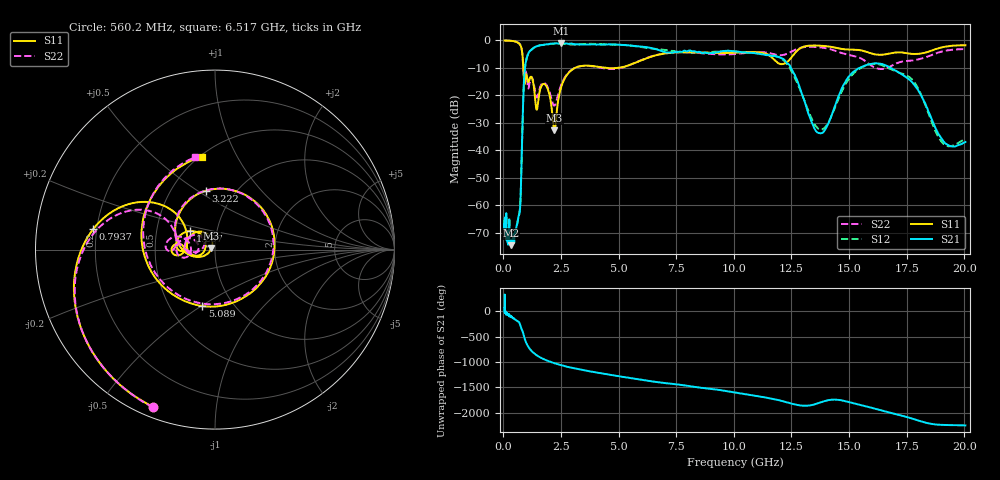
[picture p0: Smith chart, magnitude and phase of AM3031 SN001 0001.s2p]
# Hz S DB R 50
!freq MagS11 AngS11 MagS21 AngS21 MagS12 AngS12 MagS22 AngS22
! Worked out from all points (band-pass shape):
!   1601 points, 50 MHz to 20.05 GHz, reference 50 ohm
!   highest |S21| = -1.04 dB at 2.507 GHz (marker M1); lowest = -74.6 dB at 324.2 MHz (marker M2)
!   |S21| within 3 dB of the highest: 1.129 GHz to 6.924 GHz (5.795 GHz wide, 144 % of centre); 9.404 GHz to 10.13 GHz (725.5 MHz wide, 7.43 % of centre)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
!   lowest |S11| = -32.7 dB at 2.207 GHz (marker M3), VSWR 1.05, Z = 47.9 + j0.854 ohm
!   |S11| at or under -10 dB: 862.9 MHz to 3.104 GHz (2.241 GHz wide, 113 % of centre); 4.461 GHz to 4.944 GHz (483.7 MHz wide, 10.3 % of centre)
!   |S22| runs from -23.8 to 0.0 dB; largest |S21 - S12| = 0.067
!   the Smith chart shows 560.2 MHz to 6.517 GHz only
!   S11 on the Smith chart (normalised r, x): 560.2 MHz: 0.04, -0.68; 793.7 MHz: 0.19, +0.08; 1.287 GHz: 0.74, +0.16; 3.222 GHz: 0.73, +0.54; 5.089 GHz: 0.72, -0.50; 6.517 GHz: 0.51, +0.73
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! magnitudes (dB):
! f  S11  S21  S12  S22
! 50 MHz  0.0  -65.7  -67.0  0.0
! 135.9 MHz  0.0  -69.9  -71.4  0.0
! 324.2 MHz  -0.1  -74.6  -74.2  -0.1
! 369.6 MHz  -0.2  -73.3  -73.5  -0.2
! 560.2 MHz  -0.5  -68.0  -68.1  -0.5
! 717.4 MHz  -1.5  -61.5  -61.1  -1.5
! 793.7 MHz  -3.2  -41.7  -41.4  -3.4
! 888.1 MHz  -14.4  -15.1  -15.1  -13.1
! 1.005 GHz  -12.6  -6.6  -6.5  -12.8
! 1.287 GHz  -15.2  -2.8  -2.9  -14.6
! 1.879 GHz  -16.9  -1.5  -1.5  -16.4
! 2.207 GHz  -32.7  -1.1  -1.1  -23.8
! 2.507 GHz  -16.9  -1.0  -1.1  -16.2
! 2.722 GHz  -13.0  -1.1  -1.3  -12.7
! 3.222 GHz  -9.6  -1.4  -1.4  -9.6
! 5.089 GHz  -9.8  -1.6  -1.6  -10.0
! 6.517 GHz  -5.6  -3.0  -3.0  -5.6
! 7.402 GHz  -4.4  -4.3  -3.9  -4.4
! 11.91 GHz  -8.2  -6.0  -5.9  -5.3
! 13.73 GHz  -1.9  -33.8  -32.4  -2.5
! 16.44 GHz  -5.2  -8.6  -9.1  -10.4
! 20.05 GHz  -1.8  -37.0  -35.9  -3.1
